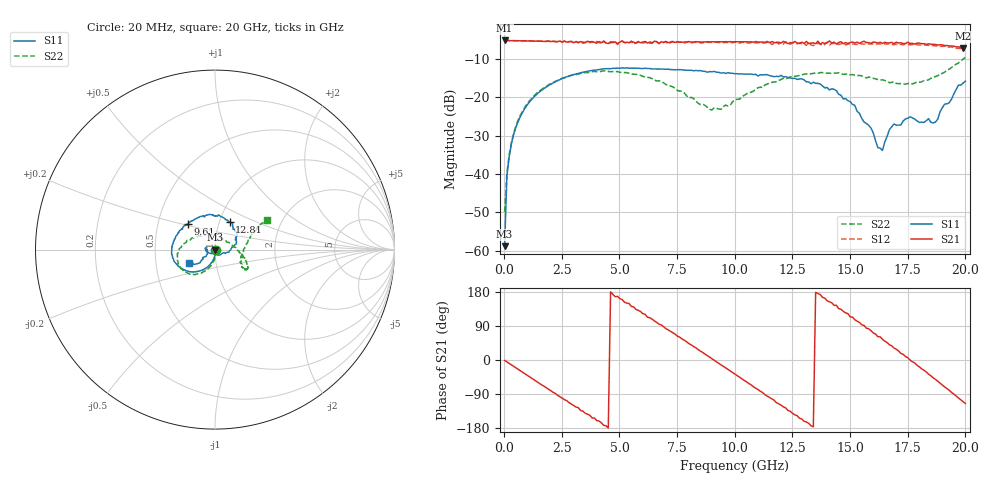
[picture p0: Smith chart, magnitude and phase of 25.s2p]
!Agilent Technologies,N5230A,US43500223,A.07.50.48
!Agilent N5230A: A.07.50.48
!Date: Wednesday, September 16, 2015 12:37:19
!Correction: S11(Full 2 Port(1,2))
!S21(Full 2 Port(1,2))
!S12(Full 2 Port(1,2))
!S22(Full 2 Port(1,2))
!S2P File: Measurements: S11, S21, S12, S22:
# Hz S  dB  R 50
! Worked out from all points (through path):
!   201 points, 20 MHz to 20 GHz, reference 50 ohm
!   highest |S21| = -5.12 dB at 20 MHz (marker M1); lowest = -7.1 dB at 19.9 GHz (marker M2)
!   group delay of S21, straight-line fit = 114 ps
!   lowest |S11| = -58.8 dB at 20 MHz (marker M3), VSWR 1.00, Z = 50.1 - j0.101 ohm
!   |S11| at or under -10 dB: start of sweep to end of sweep
!   |S22| runs from -49.9 to -9.5 dB; largest |S21 - S12| = 0.075
!   S11 on the Smith chart (normalised r, x): 20 MHz: 1.00, -0.00; 9.61 GHz: 0.71, +0.21; 12.81 GHz: 1.12, +0.36; 20 GHz: 0.74, -0.11
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2e7  -58.84 -61.6  -5.12 -1.0  -5.12 -0.9  -49.86 -16.5
1.199e8  -40.39 -76.9  -5.14 -5.1  -5.14 -5.1  -39.76 -66.8
3.197e8  -31.99 -87.0  -5.18 -13.1  -5.17 -13.2  -31.59 -81.8
6.194e8  -26.07 -97.0  -5.20 -25.1  -5.20 -25.3  -25.72 -92.3
2.1179e9  -16.21 -128.4  -5.37 -85.1  -5.25 -84.9  -16.06 -122.0
3.4166e9  -13.40 -150.5  -5.56 -135.1  -5.91 -136.5  -13.53 -143.2
5.1149e9  -12.28 -174.1  -5.24 159.6  -5.28 158.3  -13.46 -171.0
6.7133e9  -12.53 169.7  -5.92 94.7  -5.94 92.3  -15.62 162.3
8.4116e9  -13.02 153.5  -5.50 27.6  -5.45 24.3  -21.53 116.2
9.6104e9  -13.74 136.6  -5.44 -20.9  -5.68 -23.4  -21.98 42.4
1.001e10  -13.81 129.0  -5.45 -37.3  -5.55 -39.6  -20.59 21.2
1.14086e10  -14.04 99.3  -5.36 -95.4  -5.61 -97.5  -16.52 -10.4
1.28072e10  -15.17 62.1  -5.86 -153.6  -5.84 -153.8  -14.24 -24.1
1.34066e10  -16.03 45.9  -5.73 -176.2  -6.45 179.4  -13.70 -27.8
1.4006e10  -17.38 28.1  -5.69 156.2  -5.58 155.8  -13.70 -31.2
1.53047e10  -23.63 -14.1  -5.56 102.6  -6.17 101.8  -14.27 -35.0
1.64036e10  -33.86 -120.1  -5.89 54.6  -6.07 52.0  -15.40 -28.5
1.67033e10  -28.43 -149.8  -5.75 40.3  -6.03 39.2  -16.15 -26.4
1.8002e10  -26.52 173.5  -5.80 -18.0  -6.32 -20.8  -16.03 -1.9
1.87013e10  -26.43 -151.5  -6.18 -51.0  -6.52 -54.2  -14.52 13.2
1.99001e10  -16.27 -150.4  -7.13 -110.0  -7.45 -114.9  -10.00 28.8
2e10  -15.75 -152.8  -6.95 -115.0  -7.55 -120.4  -9.52 29.1
